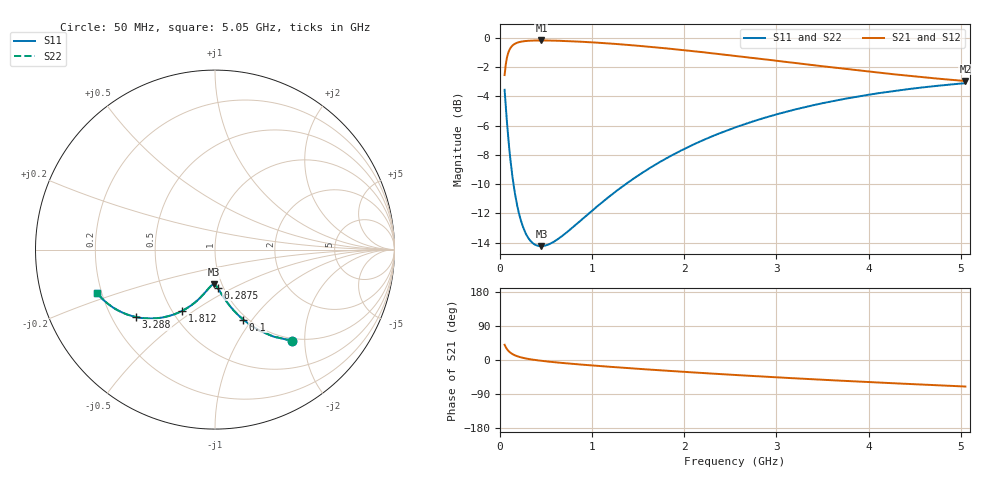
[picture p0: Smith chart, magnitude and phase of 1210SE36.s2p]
! AVX Thin Film Operation		Date: August 2001
! Description: Accu-P® Series, Thin Film, SMD, RF Capacitor
! Part Number: 12101J360FBT
! 50 MHz  -  5.05 GHz
! Serial Measurements
# mhz S db R 50
!	S11		S21		S12		S22
!	dB	Phase	dB	Phase	dB	Phase	dB	Phase
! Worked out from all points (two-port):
!   401 points, 50 MHz to 5.05 GHz, reference 50 ohm
!   highest |S21| = -0.17 dB at 450 MHz (marker M1); lowest = -2.9 dB at 5.05 GHz (marker M2)
!   |S21| within 3 dB of the highest: start of sweep to end of sweep
!   lowest |S11| = -14.2 dB at 450 MHz (marker M3), VSWR 1.48, Z = 45.8 - j18.4 ohm
!   |S11| at or under -10 dB: 146.4 MHz to 1.364 GHz (1.218 GHz wide, 161 % of centre)
!   |S22| runs from -14.2 to -3.1 dB; largest |S21 - S12| = 0
!   S11 on the Smith chart (normalised r, x): 50 MHz: 0.96, -1.74; 100 MHz: 0.95, -0.90; 287.5 MHz: 0.94, -0.42; 1.812 GHz: 0.56, -0.45; 3.288 GHz: 0.30, -0.34; 5.05 GHz: 0.18, -0.17
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50  -3.54 -49.8  -2.54 40.2  -2.54 40.2  -3.54 -49.8
75  -5.74 -61.1  -1.35 28.9  -1.35 28.9  -5.74 -61.1
87.5  -6.68 -65.0  -1.05 25.0  -1.05 25.0  -6.68 -65.0
100  -7.54 -68.1  -0.84 21.8  -0.84 21.8  -7.54 -68.1
112.5  -8.31 -70.7  -0.69 19.3  -0.69 19.3  -8.31 -70.7
137.5  -9.61 -74.7  -0.50 15.2  -0.50 15.2  -9.61 -74.7
187.5  -11.49 -80.1  -0.32 9.9  -0.32 9.9  -11.49 -80.1
237.5  -12.71 -83.6  -0.24 6.3  -0.24 6.3  -12.71 -83.6
287.5  -13.48 -86.2  -0.20 3.7  -0.20 3.7  -13.48 -86.2
362.5  -14.07 -89.3  -0.17 0.7  -0.17 0.7  -14.07 -89.3
450  -14.25 -92.1  -0.17 -2.1  -0.17 -2.1  -14.25 -92.1
612.5  -13.83 -96.3  -0.18 -6.4  -0.18 -6.4  -13.83 -96.3
887.5  -12.43 -102.2  -0.26 -12.2  -0.26 -12.2  -12.43 -102.2
1275  -10.41 -109.3  -0.42 -19.4  -0.42 -19.4  -10.41 -109.3
1725  -8.52 -116.9  -0.66 -27.0  -0.66 -27.0  -8.52 -116.9
1812.5  -8.21 -118.3  -0.71 -28.4  -0.71 -28.4  -8.21 -118.3
2175  -7.07 -124.0  -0.95 -34.0  -0.95 -34.0  -7.07 -124.0
2550  -6.12 -129.5  -1.22 -39.5  -1.22 -39.5  -6.12 -129.5
3287.5  -4.76 -139.4  -1.77 -49.5  -1.77 -49.5  -4.76 -139.4
3387.5  -4.62 -140.7  -1.85 -50.7  -1.85 -50.7  -4.62 -140.7
4225  -3.67 -150.8  -2.45 -60.8  -2.45 -60.8  -3.67 -150.8
5050  -3.09 -159.9  -2.94 -70.0  -2.94 -70.0  -3.09 -160.0
